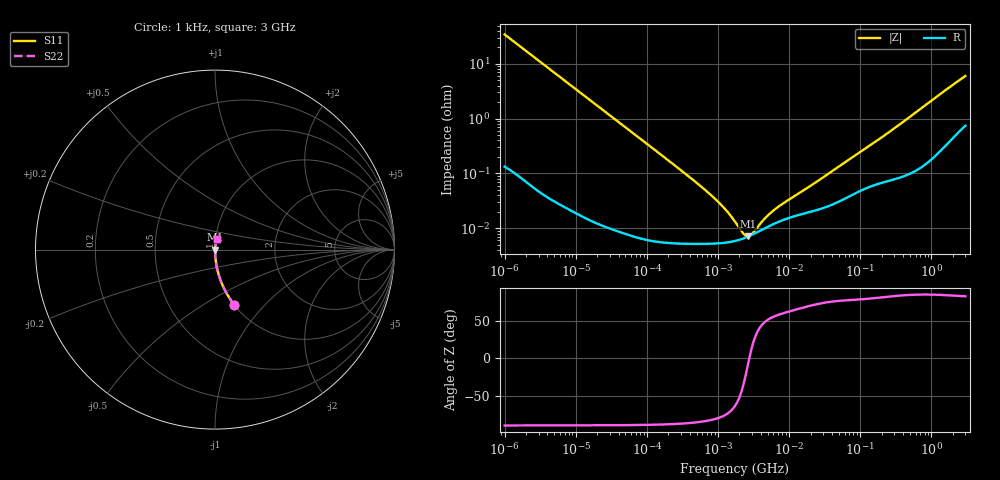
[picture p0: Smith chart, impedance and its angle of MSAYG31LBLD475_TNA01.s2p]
! MSAYG31LBLD475_TNA01  S-PARAMETER MODEL  ( Standard Model )
! Model Generated by TAIYO YUDEN Corporation (http://www.ty-top.com)
! Version 1.0
! TAIYO YUDEN Control No. 220601
! Copyright(c) 2012 TAIYO YUDEN CO.,LTD. All Rights Reserved.
! Product Description (link to TY-COMPAS)
! https://ds.yuden.co.jp/TYCOMPAS/or/detail?pn=MSAYG31LBLD475KTNA01&u=M
! Products Name : Multilayer Ceramic Capacitors
! Characteristics :
!  Capacitance : 4.7 [uF] , Rated Voltage : 35 [V] , TCC : X5R
!  Case Size : 3.2 x 1.6 / 0.126 x 0.063 [mm/inch] , Thickness : 1.6 / 0.063 [mm/inch]
!  (Conditions: Temperature = 25 [degC] , DC Bias Voltage = 0 [V])
! External Node Assignments :
!  1  o---| |---o  2
! GND o---------o GND
! Frequency Range : 1kHz  -  3GHz  [ 401 STEP ]
# MHZ S RI R 50
! Freq[MHz].  S11 Real  S11 Imag  S21 Real  S21 Imag  S12 Real  S12 Imag  S22 Real  S22 Imag
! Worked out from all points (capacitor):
!   401 points, 1 kHz to 3 GHz, reference 50 ohm
!   read as one part in series: C = 4.63 uF near 1.077 kHz
!   lowest |Z| = 7.1 mohm at 2.61 MHz (marker M1)
!   series resonance near 2.748 MHz, so ESL is about 720 pH
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0.001  0.1063 -0.3063  0.8937 0.3063  0.8937 0.3063  0.1063 -0.3063
0.001685  0.0407 -0.1955  0.9593 0.1955  0.9593 0.1955  0.0407 -0.1955
0.00306  0.0129 -0.111  0.9871 0.111  0.9871 0.111  0.0129 -0.111
0.005768  0.00383 -0.0595  0.9962 0.0595  0.9962 0.0595  0.00383 -0.0595
0.01216  0.00097 -0.0284  0.999 0.0284  0.999 0.0284  0.00097 -0.0284
0.147855  6.14e-05 -0.00234  0.9999 0.00234  0.9999 0.00234  6.14e-05 -0.00234
0.419985  5.24e-05 -0.000808  0.9999 0.000808  0.9999 0.000808  5.24e-05 -0.000808
0.791611  5.23e-05 -0.000402  0.9999 0.000402  0.9999 0.000402  5.23e-05 -0.000402
1.238299  5.43e-05 -0.000222  0.9999 0.000222  0.9999 0.000222  5.43e-05 -0.000222
1.732051  5.85e-05 -0.000118  0.9999 0.000118  0.9999 0.000118  5.85e-05 -0.000118
1.937042  6.08e-05 -8.77e-05  0.9999 8.77e-05  0.9999 8.77e-05  6.08e-05 -8.77e-05
2.087011  6.27e-05 -6.8e-05  0.9999 6.8e-05  0.9999 6.8e-05  6.27e-05 -6.8e-05
2.610246  7e-05 -1.22e-05  0.9999 1.22e-05  0.9999 1.22e-05  7e-05 -1.22e-05
3.264662  8.01e-05 4e-05  0.9999 -4e-05  0.9999 -4e-05  8.01e-05 4e-05
3.517417  8.41e-05 5.68e-05  0.9999 -5.68e-05  0.9999 -5.68e-05  8.41e-05 5.68e-05
4.919932  0.000105 0.00013  0.9999 -0.00013  0.9999 -0.00013  0.000105 0.00013
6.629817  0.000126 0.000195  0.9999 -0.000195  0.9999 -0.000195  0.000126 0.000195
21.06097  0.000204 0.000588  0.9998 -0.000588  0.9998 -0.000588  0.000204 0.000588
256.0921  0.000768 0.00566  0.9992 -0.00566  0.9992 -0.00566  0.000768 0.00566
1652.1  0.00456 0.0341  0.9954 -0.0341  0.9954 -0.0341  0.00456 0.0341
2784.426  0.00977 0.0548  0.9902 -0.0548  0.9902 -0.0548  0.00977 0.0548
3000  0.0108 0.0585  0.9892 -0.0585  0.9892 -0.0585  0.0108 0.0585
